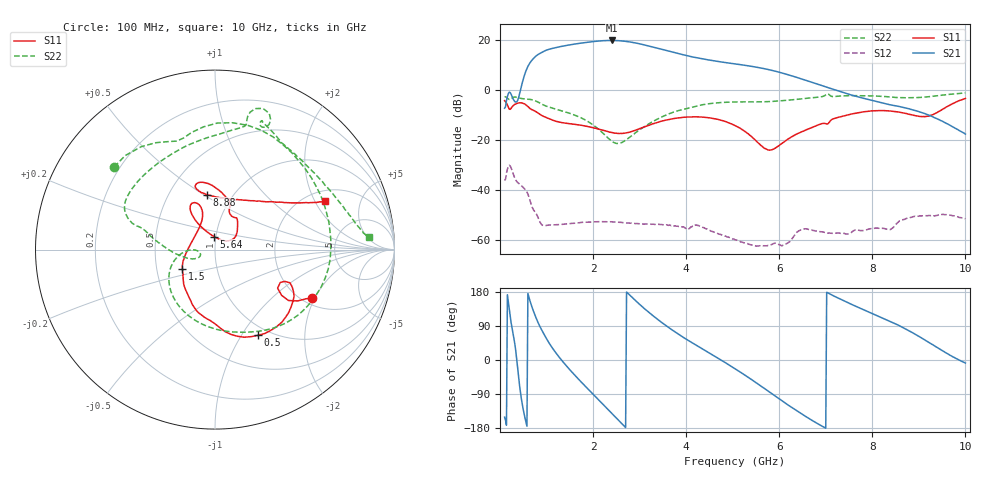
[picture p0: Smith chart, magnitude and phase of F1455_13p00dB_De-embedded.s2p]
! Integrated Device Technology
! Corporate Headquarters
! 6024 Silver Creek Valley Road
! San Jose, CA 95138  USA
! Phone:  1-408-284-8200
! Toll Free:  1-800-223-1366
! Webpage:  http://www.idt.com/
! Timing and RF Division
! 515 Groton Road, Suite 102
! Westford, MA 01886-6024
! Device:  F1455
! Description: 6-bit 0.5 dB Transmit Variable Gain Amplifier
! Frequency:  1400.0 -  2300.00 MHz
! Package:  6x6 mm Thin QFN Plastic Package: 28 pin
! State:  26
! Atten State:  13.0 dB
! Voltage:  +5.00 Volts
! Current:  217.655 mA
! Data:  The device was measured on a the F1455 evaluation board which has
!  individual transmission lines to the RF pins.  Data was collected
!  using a calibrated network analyzer.  The evaluation board was
!  de-embedded using a TRL calibration technique.
!  The reference plane is the edge of the package pin.
!  Pin  1 = CSb
!  Pin  2 = DATA
!  Pin  3 = CLK
!  Pin  4 = RSET
!  Pin  5 = GND
!  Pin  6 = RFIN  = Port 1
!  Pin  7 = GND
!  Pin  8 = NC
!  Pin  9 = NC
!  Pin 10 = NC
!  Pin 11 = NC
!  Pin 12 = NC
!  Pin 13 = NC
!  Pin 14 = /STBY
!  Pin 15 = GND
!  Pin 16 = RFOUT  = Port 2
!  Pin 17 = GND
!  Pin 18 = NC
!  Pin 19 = NC
!  Pin 20 = NC
!  Pin 21 = GND
!  Pin 22 = NC
!  Pin 23 = GND
!  Pin 24 = NC
!  Pin 25 = NC
!  Pin 26 = NC
!  Pin 27 = GND
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# GHz S dB R 50
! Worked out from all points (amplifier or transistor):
!   496 points, 100 MHz to 10 GHz, reference 50 ohm
!   highest |S21| = 19.7 dB at 2.4 GHz (marker M1)
!   |S21| within 3 dB of that: 1.164 GHz to 3.368 GHz (2.204 GHz wide, 97.3 % of centre)
!   unconditionally stable (mu >= 1): start of sweep to end of sweep
!   at 1.74 GHz: K = 23.14, MAG = 19.1 dB, |S12| = -53.0 dB
!   at 5.06 GHz: K = 98.34, MAG = 12.2 dB, |S12| = -59.9 dB
!   at 10 GHz: K = 201.37, MAG = -9.1 dB, |S12| = -51.5 dB
!   S11 on the Smith chart (normalised r, x): 100 MHz: 2.24, -1.90; 500 MHz: 0.88, -1.18; 1.5 GHz: 0.68, -0.15; 5.64 GHz: 0.98, +0.14; 8.88 GHz: 0.76, +0.51; 10 GHz: 2.47, +2.44
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0.1  -4.37 -26.5  -7.36 -150.8  -36.24 45.9  -2.78 140.7
0.38  -5.35 -40.5  -4.25 -20.4  -36.99 -114.1  -3.14 57.1
0.5  -5.45 -63.5  4.19 -130.7  -38.99 -152.0  -3.58 27.4
0.68  -7.87 -92.0  11.64 142.7  -46.24 145.6  -3.95 -14.5
0.8  -9.04 -107.4  13.84 104.0  -50.21 128.2  -4.74 -42.1
0.94  -10.64 -121.0  15.33 69.5  -54.25 124.3  -6.11 -68.3
1.22  -12.67 -139.9  16.93 15.8  -53.82 97.7  -7.84 -107.4
1.5  -13.54 -149.9  17.93 -25.7  -53.42 70.8  -9.40 -136.4
1.76  -14.20 -157.6  18.67 -59.9  -52.93 50.9  -11.35 -156.8
2.08  -15.49 -169.7  19.39 -100.2  -52.68 30.6  -15.15 -175.3
2.4  -17.05 168.6  19.69 -140.6  -52.72 12.7  -20.48 -174.9
2.58  -17.43 151.3  19.56 -163.3  -52.90 4.1  -21.34 -160.1
2.78  -16.95 132.2  19.12 172.2  -53.23 -4.5  -19.05 -154.3
3.08  -14.97 114.2  18.01 138.1  -53.64 -14.9  -14.95 -166.5
3.4  -12.91 108.3  16.53 106.0  -53.75 -26.1  -11.57 179.2
4.1  -10.84 114.6  13.25 47.6  -54.77 -44.1  -7.14 163.3
5.06  -14.33 123.6  10.30 -23.7  -59.95 -86.0  -4.86 148.3
5.64  -22.73 94.6  8.57 -71.5  -62.22 -81.7  -4.80 125.2
6.7  -15.07 44.7  3.02 -158.9  -55.99 -132.8  -3.20 78.5
8.36  -8.44 106.3  -5.91 102.9  -55.81 159.9  -2.82 62.5
8.88  -10.20 98.6  -8.08 71.0  -50.64 143.4  -3.18 42.0
10  -3.45 23.9  -17.68 -7.9  -51.50 67.8  -1.28 4.6
